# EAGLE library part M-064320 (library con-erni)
26 pol. male SMC CONNECTOR vertical , type Q, low profile Source: http://www.erni.com/DB/PDF-Drawing/SMC/064320.pdf
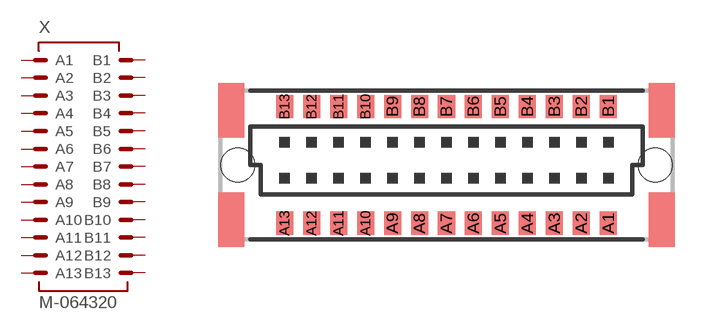
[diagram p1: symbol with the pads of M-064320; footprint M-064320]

Designator prefix X

## M-064320 (OC_FARNELL: unknown; OC_NEWARK: unknown)  [M-064320]
A1  A1  pas
A2  A2  pas
A3  A3  pas
A4  A4  pas
A5  A5  pas
A6  A6  pas
A7  A7  pas
A8  A8  pas
A9  A9  pas
A10  A10  pas
A11  A11  pas
A12  A12  pas
A13  A13  pas
B1  B1  pas
B2  B2  pas
B3  B3  pas
B4  B4  pas
B5  B5  pas
B6  B6  pas
B7  B7  pas
B8  B8  pas
B9  B9  pas
B10  B10  pas
B11  B11  pas
B12  B12  pas
B13  B13  pas

## Footprint M-064320 (pad centres in mm)
26 pol. male SMC CONNECTOR vertical , type Q, low profile Source: http://www.erni.com/DB/PDF-Drawing/SMC/064320.pdf
smd 0.8 x 1.1: A1 7.62,-2.75; A2 6.35,-2.75; A3 5.08,-2.75; A4 3.81,-2.75; A5 2.54,-2.75; A6 1.27,-2.75; A7 0,-2.75; A8 -1.27,-2.75; A9 -2.54,-2.75; A10 -3.81,-2.75; A11 -5.08,-2.75; A12 -6.35,-2.75; A13 -7.62,-2.75; B1 7.62,2.75; B2 6.35,2.75; B3 5.08,2.75; B4 3.81,2.75; B5 2.54,2.75; B6 1.27,2.75; B7 0,2.75; B8 -1.27,2.75; B9 -2.54,2.75; B10 -3.81,2.75; B11 -5.08,2.75; B12 -6.35,2.75; B13 -7.62,2.75
hole 1.6 at 9.83,0
hole 1.6 at -9.83,0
